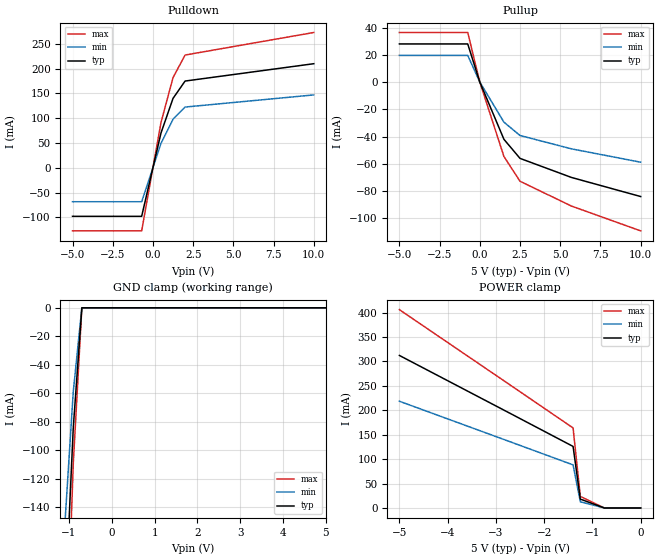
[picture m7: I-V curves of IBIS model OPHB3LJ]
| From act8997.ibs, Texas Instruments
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[Model]   OPHB3LJ
| 24-mA 3-state CMOS/TTL output buffer with 0.125 di/dt and active-low enable
| OP (97318 ALEY)
| BP (97318 ALEY)
Model_type   3-state
Polarity   Non-Inverting
| Signals   DTMS1-4
| variable   typ   min   max
C_comp   10pF   NA   NA
| variable   typ   min   max
[Voltage range]   5.0V   4.5V   5.5V
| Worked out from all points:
|   slope of the pulldown table from 0 to 0.75 V, typ, clamps not added: 8.04 ohm
|   slope of the pullup table from 0 to 0.75 V, typ, clamps not added: 35.7 ohm
|   GND clamp passes 1 mA (typ) near -0.70 V on its own axis
[pullup]
|   50C:5V:   100C:4.5V:weak  0C:5.5V:strong
| Voltage   I(typ)   I(min)   I(max)
-5V       28mA       19.6mA     36.4mA
-2.75V    28mA       19.6mA     36.4mA
-1.4V     28mA       19.6mA     36.4mA
-1.25V    28mA       19.6mA     36.4mA
-750mV    28mA       19.6mA     36.4mA
0V        0A         0A         0A
1.5V      -42mA      -29.4mA    -54.6mA
2.5V      -56mA      -39.2mA    -72.8mA
5.7V      -70mA      -49mA      -91mA
10V       -84mA      -58.8mA    -109.2mA
[pulldown]
|   50C:5V:   100C:4.5V:weak  0C:5.5V:strong
| Voltage   I(typ)   I(min)   I(max)
-5V       -98mA      -68.6mA    -127.4mA
-900mV    -98mA      -68.6mA    -127.4mA
-700mV    -98mA      -68.6mA    -127.4mA
-500mV    -70mA      -49mA      -91mA
0V        0A         0A         0A
500mV     70mA       49mA       91mA
1.25V     140mA      98mA       182mA
2V        175mA      122.5mA    227.5mA
10V       210mA      147mA      273mA
[power_clamp]
|   50C:5V:   100C:4.5V:weak  0C:5.5V:strong
| Voltage   I(typ)   I(min)   I(max)
-5V       312.2mA    218.5mA    405.9mA
-2.75V    196mA      137.2mA    254.8mA
-1.4V     126mA      88.2mA     163.8mA
-1.25V    18.2mA     12.7mA     23.7mA
-750mV    0A         0A         0A
0V        0A         0A         0A
[gnd_clamp]
|   50C:5V:   100C:4.5V:weak  0C:5.5V:strong
| Voltage   I(typ)   I(min)   I(max)
-5V       -2.8A      -2A        -3.6A
-900mV    -84mA      -58.8mA    -109.2mA
-700mV    0A         0A         0A
0V        0A         0A         0A
5V        0A         0A         0A
[ramp]
| variable   typ   min   max
dV/dt_r   1.5/2.25e-9   1.2/3.375e-9   1.8/1.5e-9
dV/dt_f   2.5/3e-9   2.1/4.5e-9   2.9/2e-9
